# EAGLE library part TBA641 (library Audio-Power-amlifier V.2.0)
http://www.datasheetcatalog.com/datasheets_pdf/T/B/A/6/TBA641.shtml
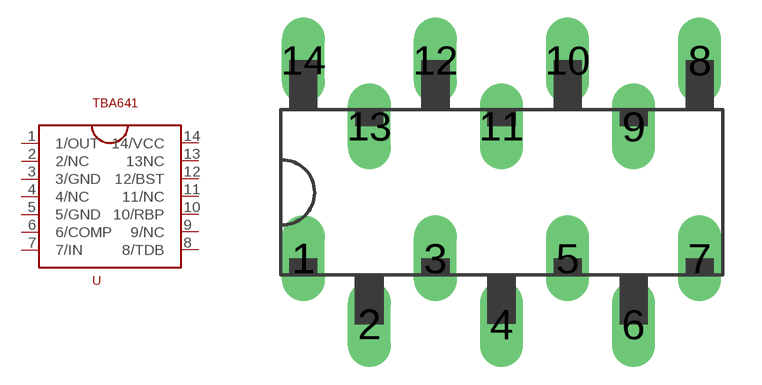
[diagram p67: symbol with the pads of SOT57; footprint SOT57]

Designator prefix -

## TBA641  [SOT57]
1  1/OUT  out
2  2/NC  nc
3  3/GND  pwr
4  4/NC  nc
5  5/GND  pwr
6  6/COMP
7  7/IN  in
8  8/TDB
9  9/NC  nc
10  10/RBP
11  11/NC  nc
12  12/BST
13  13NC  nc
14  14/VCC  pwr

## Footprint SOT57 (pad centres in mm)
drill 1.1 long: 1 -7.62,-2.54; 2 -5.08,-5.08; 3 -2.54,-2.54; 4 0,-5.08; 5 2.54,-2.54; 6 5.08,-5.08; 7 7.62,-2.54; 8 7.62,5.08; 9 5.08,2.54; 10 2.54,5.08; 11 0,2.54; 12 -2.54,5.08; 13 -5.08,2.54; 14 -7.62,5.08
